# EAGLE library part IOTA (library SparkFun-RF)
SparkFun IOTA - Integrated Open-source Transceiver for ARGOS
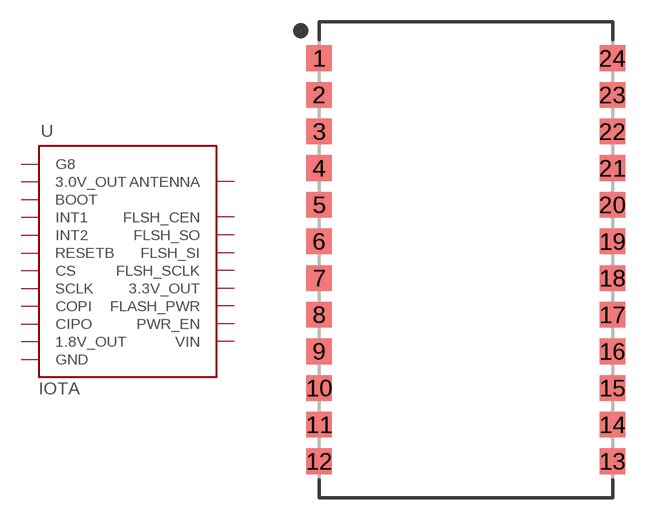
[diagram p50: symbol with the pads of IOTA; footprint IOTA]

Designator prefix -

## IOTA (PROD_ID: SUB-15839)  [IOTA]
1  G8  in
2  3.0V_OUT  out
3  BOOT  in
4  INT1  out
5  INT2  out
6  RESETB  in
7  CS  in
8  SCLK  in
9  COPI  in
10  CIPO  out
11  1.8V_OUT  out
12  GND  pwr
13  GND  pwr
14  VIN  pwr
15  PWR_EN  in
16  FLASH_PWR  in
17  3.3V_OUT  out
18  FLSH_SCLK  out
19  FLSH_SI  out
20  FLSH_SO  in
21  FLSH_CEN  out
22  GND  pwr
23  ANTENNA
24  GND  pwr

## Footprint IOTA (pad centres in mm)
ARTIC R2 Module
smd 1.778 x 1.778: 1 -10.16,13.97; 2 -10.16,11.43; 3 -10.16,8.89; 4 -10.16,6.35; 5 -10.16,3.81; 6 -10.16,1.27; 7 -10.16,-1.27; 8 -10.16,-3.81; 9 -10.16,-6.35; 10 -10.16,-8.89; 11 -10.16,-11.43; 12 -10.16,-13.97; 13 10.16,-13.97; 14 10.16,-11.43; 15 10.16,-8.89; 16 10.16,-6.35; 17 10.16,-3.81; 18 10.16,-1.27; 19 10.16,1.27; 20 10.16,3.81; 21 10.16,6.35; 22 10.16,8.89; 23 10.16,11.43; 24 10.16,13.97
